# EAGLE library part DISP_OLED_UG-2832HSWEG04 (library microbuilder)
128x32 SPI 0.91" Monochrome OLED Display
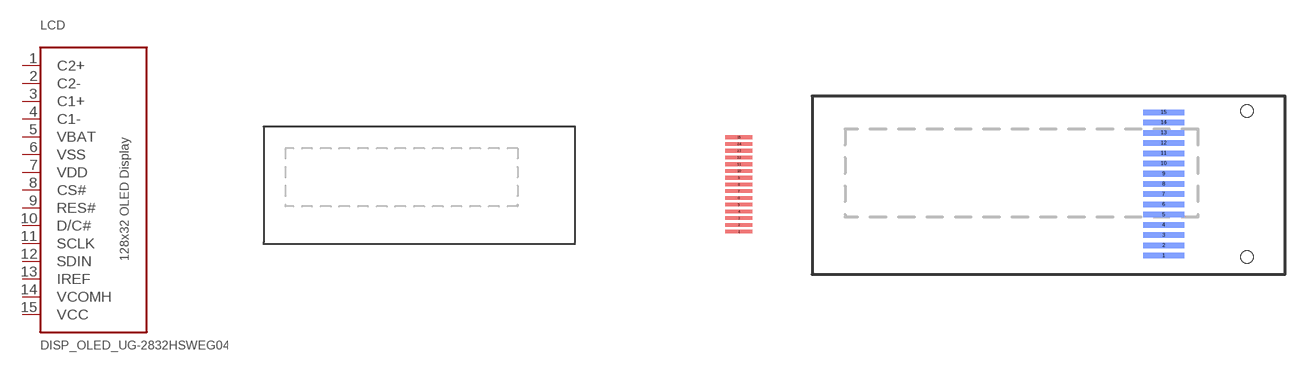
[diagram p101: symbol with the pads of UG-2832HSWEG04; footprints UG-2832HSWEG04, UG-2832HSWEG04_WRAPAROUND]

Designator prefix LCD

## DISP_OLED_UG-2832HSWEG04  [UG-2832HSWEG04]
1  C2+
2  C2-
3  C1+
4  C1-
5  VBAT
6  VSS
7  VDD
8  CS#
9  RES#
10  D/C#
11  SCLK
12  SDIN
13  IREF
14  VCOMH
15  VCC

## DISP_OLED_UG-2832HSWEG04WRAPAROUND  [UG-2832HSWEG04_WRAPAROUND]
Pads as for UG-2832HSWEG04

## Footprint UG-2832HSWEG04 (pad centres in mm)
128x32 OLED Display - 0.91" (30x11.5mm)
smd 2.6 x 0.35: 1 15.8,-4.55; 2 15.8,-3.9; 3 15.8,-3.25; 4 15.8,-2.6; 5 15.8,-1.95; 6 15.8,-1.3; 7 15.8,-0.65; 8 15.8,0; 9 15.8,0.65; 10 15.8,1.3; 11 15.8,1.95; 12 15.8,2.6; 13 15.8,3.25; 14 15.8,3.9; 15 15.8,4.55

## Footprint UG-2832HSWEG04_WRAPAROUND (pad centres in mm)
smd 2.6 x 0.35 bottom: 1 -7.7,-4.55; 2 -7.7,-3.9; 3 -7.7,-3.25; 4 -7.7,-2.6; 5 -7.7,-1.95; 6 -7.7,-1.3; 7 -7.7,-0.65; 8 -7.7,0; 9 -7.7,0.65; 10 -7.7,1.3; 11 -7.7,1.95; 12 -7.7,2.6; 13 -7.7,3.25; 14 -7.7,3.9; 15 -7.7,4.55
hole 0.8 at -2.4,4.625
hole 0.8 at -2.4,-4.625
